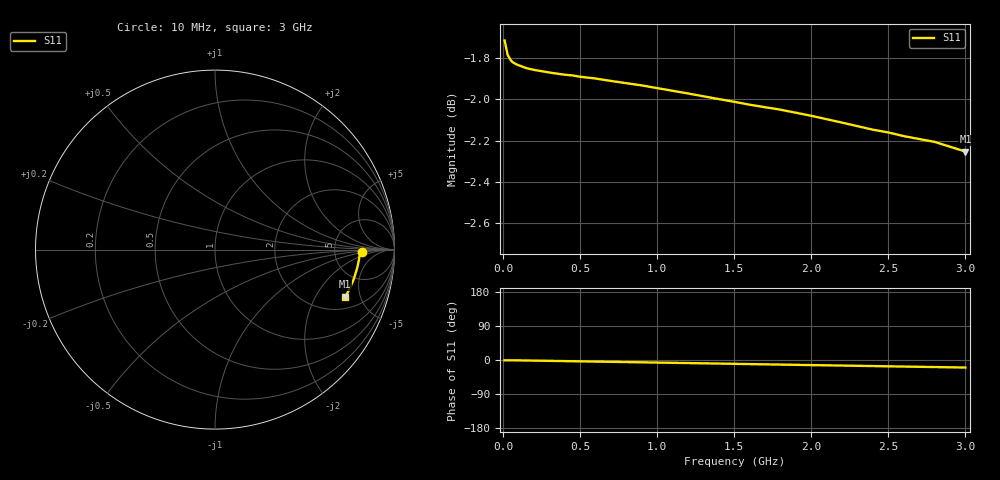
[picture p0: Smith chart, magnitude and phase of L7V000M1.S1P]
! SIEMENS Small Signal Semiconductors
! BAR14-1
! Si PIN Diode in SOT23
! IF = 0.1 mA
! S-Parameters:  July  1992
# GHz  S  MA  R  50
!  f  S11
! GHz  MAG  ANG
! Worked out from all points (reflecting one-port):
!   31 points, 10 MHz to 3 GHz, reference 50 ohm
!   lowest |S11| = -2.3 dB at 3 GHz (marker M1), VSWR 7.75, Z = 140 - j182 ohm
!   phase of S11 starts at -1 deg and turns -19 deg over the sweep
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0.01  0.821 -0.8
0.03  0.8143 -0.8
0.05  0.812 -0.8
0.06  0.8112 -0.8
0.08  0.8103 -0.9
0.1  0.8097 -1.0
0.15  0.8084 -1.3
0.3  0.8064 -2.2
0.35  0.8059 -2.6
0.4  0.8054 -2.9
0.45  0.8051 -3.2
0.5  0.8045 -3.5
0.6  0.8037 -4.2
0.7  0.8026 -4.8
0.8  0.8016 -5.5
0.9  0.8006 -6.1
1  0.7994 -6.8
1.2  0.797 -8.1
1.4  0.7945 -9.4
1.6  0.792 -10.8
1.8  0.7898 -12.1
2  0.7871 -13.4
2.2  0.7841 -14.7
2.4  0.781 -16.0
2.5  0.7798 -16.7
2.6  0.7782 -17.3
2.8  0.7757 -18.6
3  0.7715 -19.9
